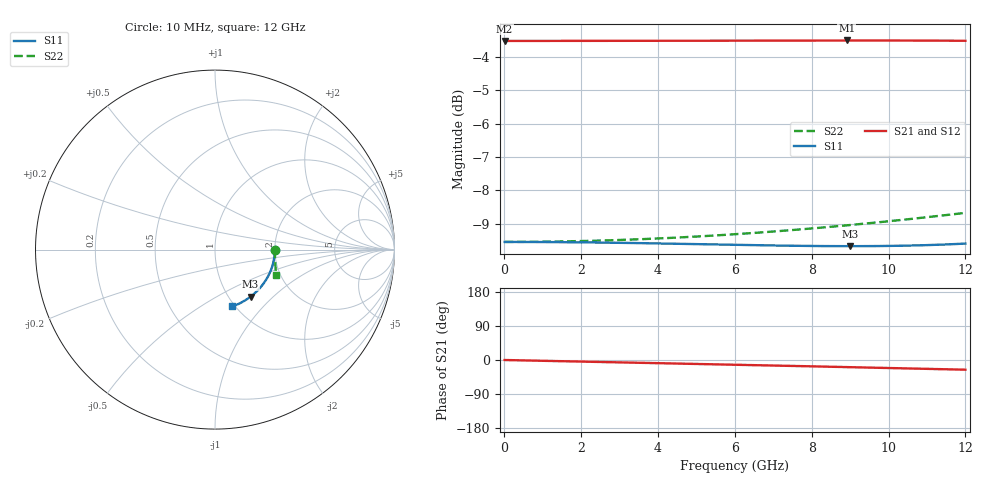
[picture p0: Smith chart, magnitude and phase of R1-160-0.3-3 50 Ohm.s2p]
!version-2
!date-03.2021
# MHz S RI R 50
!Freq ReS11 ImS11 ReS21 ImS21 ReS12 ImS12 ReS22 ImS22
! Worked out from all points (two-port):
!   601 points, 10 MHz to 12 GHz, reference 50 ohm
!   highest |S21| = -3.51 dB at 8.91 GHz (marker M1); lowest = -3.5 dB at 10 MHz (marker M2)
!   |S21| within 3 dB of the highest: start of sweep to end of sweep
!   lowest |S11| = -9.7 dB at 9.01 GHz (marker M3), VSWR 1.98, Z = 62.7 - j36.8 ohm
!   |S11| at or under -10 dB: nowhere
!   |S22| runs from -9.5 to -8.7 dB; largest |S21 - S12| = 0
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10  0.3333 -0.000323  0.6667 -0.000239  0.6667 -0.000239  0.3333 -0.00011
70  0.3333 -0.00226  0.6667 -0.00167  0.6667 -0.00167  0.3333 -0.000773
1010  0.3316 -0.0326  0.6663 -0.0241  0.6663 -0.0241  0.3334 -0.0112
1510  0.3295 -0.0486  0.6658 -0.0361  0.6658 -0.0361  0.3335 -0.0167
2010  0.3265 -0.0646  0.665 -0.048  0.665 -0.048  0.3336 -0.0222
2510  0.3227 -0.0805  0.6641 -0.06  0.6641 -0.06  0.3338 -0.0278
3010  0.3181 -0.0962  0.663 -0.072  0.663 -0.072  0.3339 -0.0334
3510  0.3126 -0.1117  0.6617 -0.084  0.6617 -0.084  0.3341 -0.039
4010  0.3063 -0.127  0.6601 -0.096  0.6601 -0.096  0.3344 -0.0447
4510  0.2992 -0.1421  0.6584 -0.108  0.6584 -0.108  0.3346 -0.0504
5010  0.2912 -0.157  0.6564 -0.12  0.6564 -0.12  0.3349 -0.0561
5510  0.2824 -0.1715  0.6542 -0.132  0.6542 -0.132  0.3352 -0.0619
6010  0.2728 -0.1857  0.6517 -0.1441  0.6517 -0.1441  0.3356 -0.0677
6510  0.2624 -0.1995  0.649 -0.1561  0.649 -0.1561  0.3359 -0.0736
7010  0.2511 -0.2129  0.6461 -0.1682  0.6461 -0.1682  0.3363 -0.0796
8010  0.2263 -0.2384  0.6395 -0.1923  0.6395 -0.1923  0.337 -0.0916
8910  0.2012 -0.2597  0.6326 -0.214  0.6326 -0.214  0.3377 -0.1028
9010  0.1983 -0.2619  0.6317 -0.2165  0.6317 -0.2165  0.3377 -0.104
10010  0.1673 -0.283  0.6229 -0.2405  0.6229 -0.2405  0.3384 -0.1167
11050  0.132 -0.3022  0.6124 -0.2655  0.6124 -0.2655  0.3391 -0.1303
11590  0.1124 -0.3109  0.6064 -0.2784  0.6064 -0.2784  0.3394 -0.1375
12000  0.0971 -0.3169  0.6016 -0.2881  0.6016 -0.2881  0.3396 -0.143
